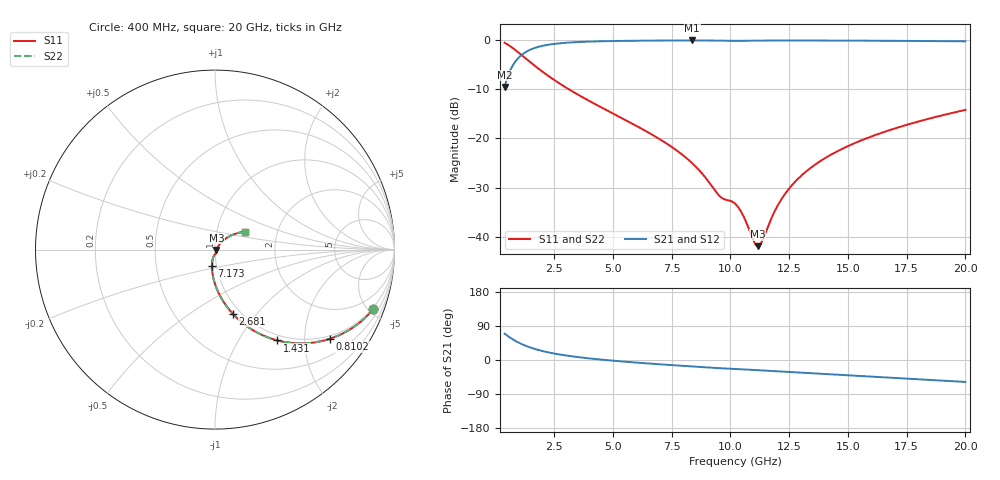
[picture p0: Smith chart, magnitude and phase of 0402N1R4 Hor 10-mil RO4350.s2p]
# GHz S MA R 50
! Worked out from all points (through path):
!   1960 points, 400 MHz to 20 GHz, reference 50 ohm
!   highest |S21| = -0.05 dB at 8.384 GHz (marker M1); lowest = -9.5 dB at 400 MHz (marker M2)
!   group delay of S21, straight-line fit = 12.9 ps
!   lowest |S11| = -41.9 dB at 11.18 GHz (marker M3), VSWR 1.02, Z = 50.8 - j0.249 ohm
!   |S11| at or under -10 dB: 3.137 GHz to end of sweep
!   |S22| runs from -41.9 to -0.5 dB; largest |S21 - S12| = 0
!   S11 on the Smith chart (normalised r, x): 400 MHz: 0.91, -5.38; 810.2 MHz: 0.91, -2.65; 1.431 GHz: 0.91, -1.48; 2.681 GHz: 0.92, -0.76; 7.173 GHz: 0.95, -0.17; 20 GHz: 1.37, +0.28
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0.4  0.9424 -20.5  0.3343 69.5  0.3343 69.5  0.9424 -20.5
0.8102093  0.8108 -37.8  0.5847 52.2  0.5847 52.2  0.8108 -37.8
1.430526  0.6133 -55.6  0.7888 34.3  0.7888 34.3  0.6133 -55.6
1.980807  0.4839 -65.7  0.8739 24.1  0.8739 24.1  0.4839 -65.7
2.681164  0.37 -74.6  0.9274 15.2  0.9274 15.2  0.37 -74.6
3.671669  0.2664 -83.1  0.962 6.5  0.962 6.5  0.2664 -83.1
6.943338  0.1002 -99.7  0.9922 -11.1  0.9922 -11.1  0.1002 -99.7
7.173456  0.09259 -100.5  0.9929 -12.1  0.9929 -12.1  0.09259 -100.5
8.384074  0.0559 -103.6  0.9947 -17.1  0.9947 -17.1  0.0559 -103.6
9.554671  0.02579 -88.4  0.9891 -21.7  0.9891 -21.7  0.02579 -88.4
10.205  0.02168 -73.6  0.9855 -23.6  0.9855 -23.6  0.02168 -73.6
10.48515  0.01753 -71.8  0.9876 -24.5  0.9876 -24.5  0.01753 -71.8
11.00541  0.008948 -42.3  0.9909 -26.3  0.9909 -26.3  0.008948 -42.3
11.1755  0.008013 -17.8  0.9916 -26.9  0.9916 -26.9  0.008013 -17.8
11.33558  0.008831 5.6  0.9921 -27.5  0.9921 -27.5  0.008831 5.6
11.84584  0.01732 39.3  0.993 -29.3  0.993 -29.3  0.01732 39.3
12.26605  0.02597 46.2  0.9933 -30.8  0.9933 -30.8  0.02597 46.2
12.80633  0.03733 48.9  0.9933 -32.7  0.9933 -32.7  0.03733 48.9
13.46667  0.05122 49.1  0.9929 -35.1  0.9929 -35.1  0.05122 49.1
14.85738  0.08047 46.5  0.9911 -39.9  0.9911 -39.9  0.08047 46.5
16.73834  0.1208 41.1  0.9869 -46.5  0.9869 -46.5  0.1208 41.1
20  0.1954 30.5  0.9744 -57.9  0.9744 -57.9  0.1954 30.5
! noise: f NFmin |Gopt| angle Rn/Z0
0.4  0.001388  0.819  4.517  0.001603
2.571  0.005184  0.6862  7.997  0.003192
4.752  0.008118  0.6396  12.71  0.004203
6.933  0.01085  0.6145  17.51  0.005117
9.104  0.01888  0.6967  22.11  0.01172
11.29  0.02375  0.7031  27.09  0.01485
13.47  0.02166  0.6322  31.82  0.01028
15.64  0.023  0.609  36.36  0.009899
17.82  0.02495  0.5986  40.77  0.01014
20  0.02713  0.5941  45.04  0.01058
